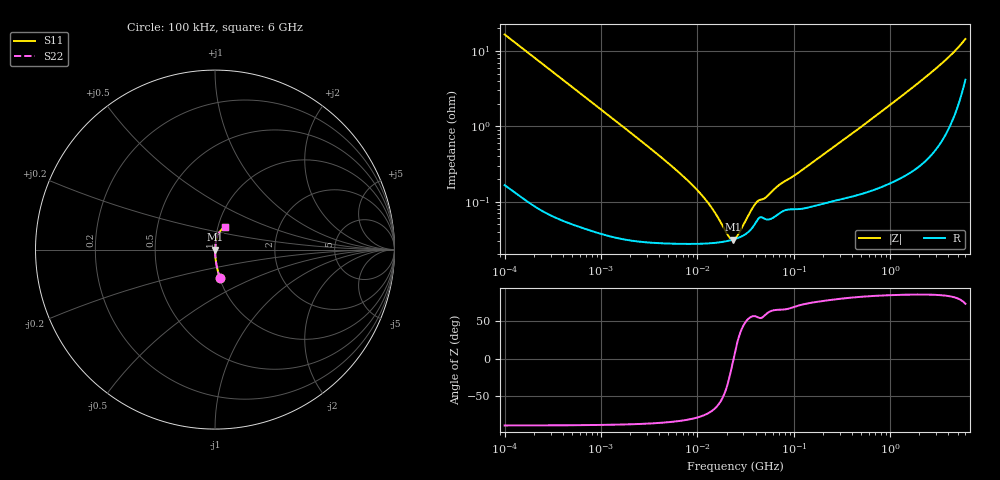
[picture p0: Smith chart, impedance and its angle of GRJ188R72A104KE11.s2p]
!Murata Part Number: GRJ188R72A104KE11
!These Parameters are Measured in Series Mode Connection
!Data Generated on Jun 19, 2026
!  o--ll--o
!Port1  Port2
!  o------o
!Operation Temp=25[degC], DC Bias Voltage=0[V]
!Freq. Start=100[kHz] Stop=6[GHz] 401[Steps]
# Hz S RI R 50
!Freq.(Hz) S11(Real) S11(Imag) S21(Real) S21(Imag) S12(Real) S12(Imag) S22(Real) S22(Imag)
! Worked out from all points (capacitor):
!   401 points, 100 kHz to 6 GHz, reference 50 ohm
!   read as one part in series: C = 96 nF near 105.7 kHz
!   lowest |Z| = 31.4 mohm at 23.18 MHz (marker M1)
!   series resonance near 23.67 MHz, so ESL is about 470 pH
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100000  0.0282 -0.1606  0.9718 0.1606  0.9718 0.1606  0.0282 -0.1606
228224  0.00606 -0.0723  0.9939 0.0723  0.9939 0.0723  0.00606 -0.0723
631452  0.00115 -0.0264  0.9989 0.0264  0.9989 0.0264  0.00115 -0.0264
3987316  0.000298 -0.0041  0.9997 0.0041  0.9997 0.0041  0.000298 -0.0041
7104501  0.00028 -0.00216  0.9997 0.00216  0.9997 0.00216  0.00028 -0.00216
1.073283e7  0.000278 -0.00125  0.9997 0.00125  0.9997 0.00125  0.000278 -0.00125
1.452491e7  0.000283 -0.000727  0.9997 0.000727  0.9997 0.000727  0.000283 -0.000727
2.076842e7  0.000302 -0.000189  0.9997 0.000189  0.9997 0.000189  0.000302 -0.000189
2.19429e7  0.000307 -0.000109  0.9997 0.000109  0.9997 0.000109  0.000307 -0.000109
2.318381e7  0.000313 -2.98e-05  0.9997 2.98e-05  0.9997 2.98e-05  0.000313 -2.98e-05
2.517799e7  0.000323 8.96e-05  0.9997 -8.96e-05  0.9997 -8.96e-05  0.000323 8.96e-05
2.734369e7  0.000337 0.00021  0.9997 -0.00021  0.9997 -0.00021  0.000337 0.00021
3.60007e7  0.000432 0.000635  0.9996 -0.000635  0.9996 -0.000635  0.000432 0.000635
4.130835e7  0.000559 0.000823  0.9994 -0.000823  0.9994 -0.000823  0.000559 0.000823
5.007898e7  0.000592 0.000947  0.9994 -0.000947  0.9994 -0.000947  0.000592 0.000947
7.160533e7  0.00071 0.00154  0.9993 -0.00154  0.9993 -0.00154  0.00071 0.00154
1.023848e8  0.000797 0.00211  0.9992 -0.00211  0.9992 -0.00211  0.000797 0.00211
1.546735e8  0.000873 0.00318  0.9991 -0.00318  0.9991 -0.00318  0.000873 0.00318
9.76689e8  0.00208 0.0188  0.9979 -0.0188  0.9979 -0.0188  0.00208 0.0188
3.016594e9  0.00848 0.0585  0.9915 -0.0585  0.9915 -0.0585  0.00848 0.0585
4.557193e9  0.0219 0.0926  0.9781 -0.0926  0.9781 -0.0926  0.0219 0.0926
6e9  0.0565 0.1251  0.9435 -0.1251  0.9435 -0.1251  0.0565 0.1251
